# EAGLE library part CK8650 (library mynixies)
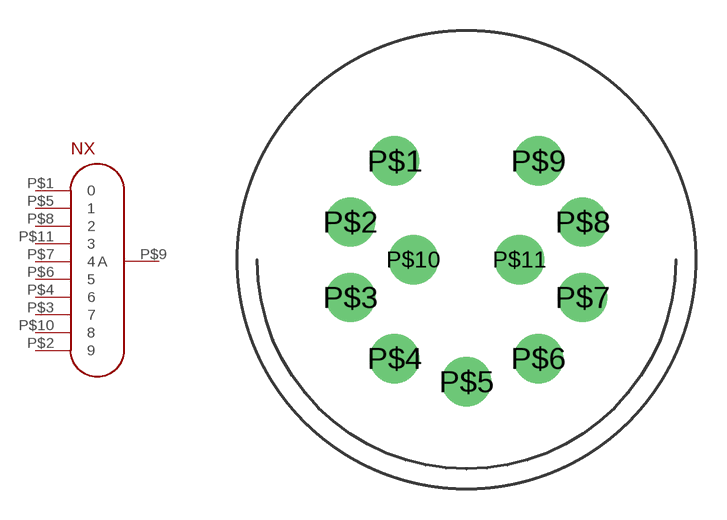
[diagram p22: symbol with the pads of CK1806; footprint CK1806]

Designator prefix NX

## CK8650D-SUB  [CK1806]
P$1  0
P$2  9
P$3  7
P$4  6
P$5  1
P$6  5
P$7  4
P$8  2
P$9  A
P$10  8
P$11  3

## Footprint CK1806 (pad centres in mm)
drill 1.6: P$1 -3.483,4.793; P$2 -5.635,1.831; P$3 -5.635,-1.831; P$4 -3.483,-4.793; P$5 0,-5.925; P$6 3.483,-4.793; P$7 5.635,-1.831; P$8 5.635,1.831; P$9 3.483,4.793; P$10 -2.58,0; P$11 2.58,0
